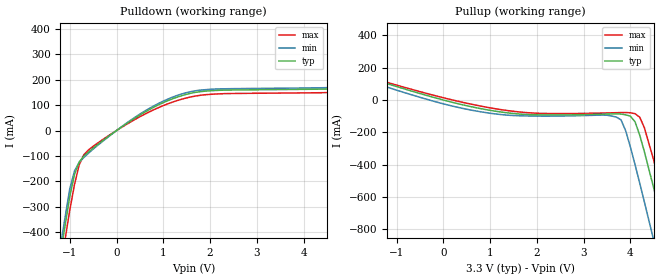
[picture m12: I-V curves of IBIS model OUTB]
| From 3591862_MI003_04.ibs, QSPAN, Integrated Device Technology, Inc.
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|   Model OUTB
[Model]   OUTB
Model_type   Output
Polarity   Non-Inverting
C_comp   5.00pF   5.00pF   5.00pF
[Voltage Range]   3.3000V   3.0000V   3.5000V
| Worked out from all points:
|   slope of the pulldown table from 0 to 0.495 V, typ, clamps not added: 8.19 ohm
|   slope of the pullup table from 0 to 0.495 V, typ, clamps not added: 14.1 ohm
[Pulldown]
| voltage   I(typ)   I(min)   I(max)
-3.3V     -3.036A    -3.001A    -3.093A
-1.5V     -828mA     -790.5mA   -888.3mA
-1V       -258.8mA   -228.6mA   -312.5mA
-900mV    -172.7mA   -159.5mA   -212.8mA
-800mV    -124.4mA   -125.2mA   -135.6mA
-600mV    -84.46mA   -89.2mA    -76.32mA
400mV     49.72mA    52.75mA    44.24mA
1.3V      131.6mA    138.2mA    118mA
5.7V      175.8mA    181.9mA    163.2mA
5.9V      218.1mA    213.5mA    220.6mA
6.1V      299.9mA    294.2mA    303mA
6.6V      528.2mA    523.9mA    528.8mA
[Pullup]
| voltage   I(typ)   I(min)   I(max)
-3.3V     344.3mA    275.4mA    443.3mA
-2.7V     237.3mA    218.7mA    239.5mA
-200mV    15.69mA    -8.13mA    28.9mA
1.6V      -86.11mA   -97.15mA   -73.04mA
3.7V      -85.54mA   -105.6mA   -78.4mA
3.9V      -91.57mA   -191mA     -77.35mA
4.1V      -134.7mA   -400.3mA   -84.49mA
4.3V      -320.5mA   -631.4mA   -171.9mA
4.5V      -545.8mA   -869.2mA   -373mA
4.7V      -780.9mA   -1.11A     -599.7mA
4.9V      -1.02A     -1.353A    -834.7mA
6.6V      -3.106A    -3.449A    -2.908A
[Ramp]
| variable   typ   min   max
dV/dt_r   1.5258/0.7847n   1.5510/0.7246n   1.4850/0.8929n
dV/dt_f   1.6988/0.7649n   1.7039/0.8648n   1.6714/0.8206n
R_load = 50.0000
| End [Model] OUTB
| End [Component] QSpan
